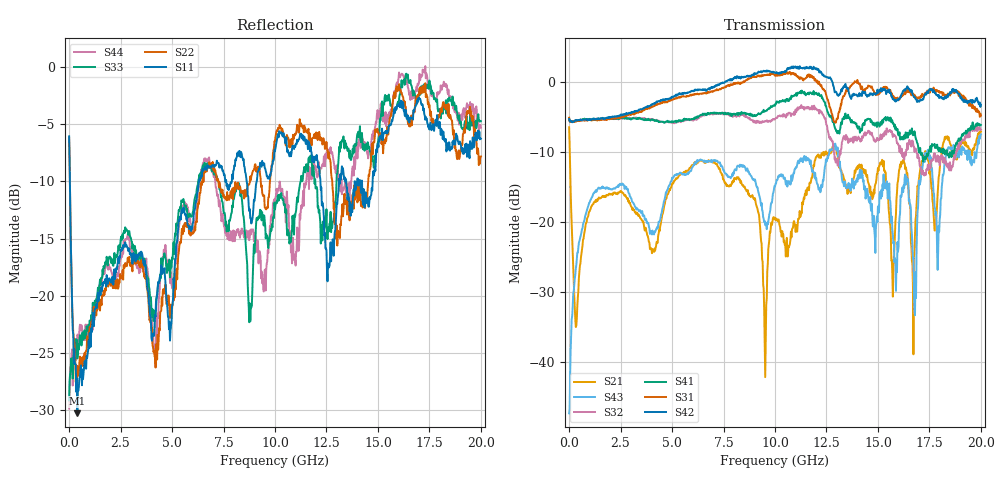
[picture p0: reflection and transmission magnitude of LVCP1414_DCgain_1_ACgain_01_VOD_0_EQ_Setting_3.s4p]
!Agilent Technologies,N5230A,MY46400459,A.07.50.48
!Agilent N5230A: A.07.50.48
!Date: Tuesday, April 17, 2012 18:46:00
!Correction: S11(Full 4 Port(1,2,3,4))
!S12(Full 4 Port(1,2,3,4))
!S13(Full 4 Port(1,2,3,4))
!S14(Full 4 Port(1,2,3,4))
!S21(Full 4 Port(1,2,3,4))
!S22(Full 4 Port(1,2,3,4))
!S23(Full 4 Port(1,2,3,4))
!S24(Full 4 Port(1,2,3,4))
!S31(Full 4 Port(1,2,3,4))
!S32(Full 4 Port(1,2,3,4))
!S33(Full 4 Port(1,2,3,4))
!S34(Full 4 Port(1,2,3,4))
!S41(Full 4 Port(1,2,3,4))
!S42(Full 4 Port(1,2,3,4))
!S43(Full 4 Port(1,2,3,4))
!S44(Full 4 Port(1,2,3,4))
!S4P File: Measurements: <S11,S12,S13,S14>,
!<S21,S22,S23,S24>,
!<S31,S32,S33,S34>,
!<S41,S42,S43,S44>:
# Hz S  dB  R 50
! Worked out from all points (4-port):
!   801 points, 300 kHz to 20 GHz, reference 50 ohm
!   strongest paths, dB at 300 kHz, 5 GHz, 10 GHz, 15 GHz, 20 GHz:
!     S42: -5.3, -2.1, 1.3, -1.3, -3.3
!     S31: -5.1, -2.6, 0.9, -1.9, -4.8
!     S41: -5.2, -5.6, -3.4, -5.8, -6.2
!     S32: -5.3, -5.8, -5.4, -8.3, -6.8
!     S43: -47.3, -13.7, -14.9, -17.8, -7.5
!     S21: -6.5, -14.5, -19.6, -12.3, -7.1
!   lowest |S11| = -30.3 dB at 400.3 MHz (marker M1), VSWR 1.06, Z = 52.9 + j1.3 ohm
!   |S11| at or under -10 dB: 37.52 MHz to 6.309 GHz (6.272 GHz wide, 198 % of centre); 8.624 GHz to 9.111 GHz (486.8 MHz wide, 5.49 % of centre); 12.21 GHz to 13.12 GHz (910.1 MHz wide, 7.19 % of centre)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
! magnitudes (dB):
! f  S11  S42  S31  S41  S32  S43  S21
! 300 kHz  -6.1  -5.3  -5.1  -5.2  -5.3  -47.3  -6.5
! 400.3 MHz  -30.3  -5.5  -5.4  -5.5  -5.5  -24.3  -31.9
! 9.925 GHz  -8.2  1.4  1.1  -3.4  -5.4  -15.8  -19.3
! 12.95 GHz  -13.7  -1.4  -5.8  -6.8  -11.5  -9.3  -9.5
! 14.03 GHz  -9.8  -2.1  -0.1  -6.7  -8.2  -13.3  -12.0
! 16.8 GHz  -3.6  -2.2  -2.0  -7.5  -9.7  -33.3  -21.7
! 20 GHz  -6.3  -3.3  -4.8  -6.2  -6.8  -7.5  -7.1
